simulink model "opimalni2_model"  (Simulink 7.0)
settings: Solver=ode45  StartTime=0.0  StopTime=10.0  RelTol=1e-3
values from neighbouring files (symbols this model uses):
  Ccit_Z1 = pol2mat(Ccit_Zp1)    [example_3_6_2_podklad.m]
  Ccit_Z2 = pol2mat(Ccit_Zp2)    [example_3_6_2_podklad.m]
  Cjmn_Z = pol2mat(Cjmn_Zp)    [example_3_6_1_podklad.m]    (also in example_3_6_2_podklad.m; example_3_6_3_podklad.m)

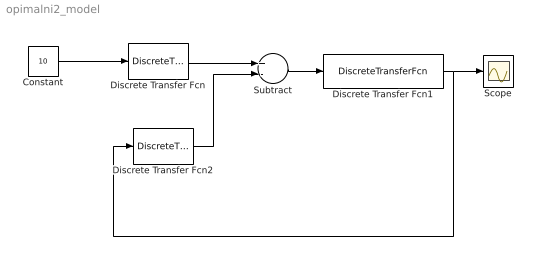
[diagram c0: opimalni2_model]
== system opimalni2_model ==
  Constant : Constant  Value=10  OutDataType=sfix(16)  OutScaling=2^0
  Discrete Transfer Fcn : DiscreteTransferFcn  Numerator=Ccit_Z1  Denominator=Cjmn_Z
  Discrete Transfer Fcn1 : DiscreteTransferFcn  Numerator=[1 -3.5 -2]  Denominator=[1 -3.5 3.5 -1]
  Discrete Transfer Fcn2 : DiscreteTransferFcn  Numerator=Ccit_Z2  Denominator=Cjmn_Z
  Scope : Scope
  Subtract : Sum  Inputs=+-  OutDataType=sfix(16)  OutScaling=2^-10
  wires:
  Discrete Transfer Fcn1/1 -> Scope/1, Discrete Transfer Fcn2/1
  Discrete Transfer Fcn/1 -> Subtract/1
  Discrete Transfer Fcn2/1 -> Subtract/2
  Subtract/1 -> Discrete Transfer Fcn1/1
  Constant/1 -> Discrete Transfer Fcn/1
